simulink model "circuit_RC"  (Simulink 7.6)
settings: Solver=ode23t  StartTime=0.0  StopTime=10.0  RelTol=1e-3
InitFcn:
  | clear all, close all
  | % Durée de la simulation
  | N=10;
  | 
  | % Hauteur de l'échelon d'entrée
  | U0=5;
  | 
  | % Valeurs de la résistance R et de la capacité C
  | R=10e3;
  | C=0.1e-3;
StopFcn:
  | close all, clc
  | load circuit_RC.mat
  | plot(x(1,:),x(2,:),x(1,:),x(3,:),x(1,:),x(4,:))
  | grid
  | title('tension d''entrée, de sortie circuit et modèle théorique')
  | xlabel('temps')
  | axis([0 N -0.2 5.2])
libraries: fl_lib x6, nesl_utility x3, elec_lib x1

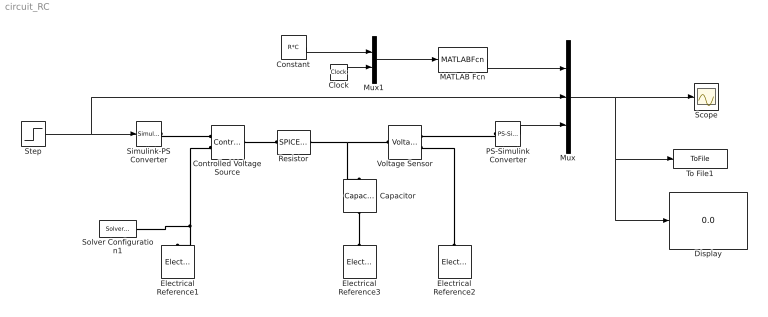
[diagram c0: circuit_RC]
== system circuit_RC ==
  Capacitor : fl_lib/Electrical/Electrical Elements/Capacitor  DialogController=NetworkEngine.DynNeDlgSource  SystemSampleTime=-1  c=C F  v0=0 V  r=0 Ohm  g=0 1/Ohm  i_Log=off  v_Log=off  vc_Log=off  LocalVarNames=|i|v|vc  LocalVarDescs=|i|v|Internal variable for voltage across capacitor term  LocalVarLogging=[0 0 0]
  Clock : Clock
  Constant : Constant  Value=R*C
  Controlled Voltage Source : fl_lib/Electrical/Electrical Sources/Controlled Voltage Source  DialogController=NetworkEngine.DynNeDlgSource  SystemSampleTime=-1  i_Log=off  v_Log=off  LocalVarNames=|current|voltage|power  LocalVarDescs=|Current (A)|Voltage (V)|Power (W)  LocalVarLogging=[0 0 0]
  Display : Display
  Electrical Reference1 : fl_lib/Electrical/Electrical Elements/Electrical Reference  DialogController=NetworkEngine.DynNeDlgSource  SystemSampleTime=-1  i_Log=off  LocalVarNames=|i  LocalVarDescs=|i  LocalVarLogging=0
  Electrical Reference2 : fl_lib/Electrical/Electrical Elements/Electrical Reference  DialogController=NetworkEngine.DynNeDlgSource  SystemSampleTime=-1  i_Log=off  LocalVarNames=|i  LocalVarDescs=|i  LocalVarLogging=0
  Electrical Reference3 : fl_lib/Electrical/Electrical Elements/Electrical Reference  DialogController=NetworkEngine.DynNeDlgSource  SystemSampleTime=-1  i_Log=off  LocalVarNames=|i  LocalVarDescs=|i  LocalVarLogging=0
  MATLAB Fcn : MATLABFcn  MATLABFcn=U0*(1-exp(-u(2)/u(1)))  Output1D=off
  Mux : Mux  Inputs=3
  Mux1 : Mux  Inputs=2
  PS-Simulink Converter : nesl_utility/PS-Simulink Converter  DialogController=NetworkEngine.DynNeUtilDlgSource  SystemSampleTime=-1  PhysicalDomain=network_engine_domain  LeftPortType=input  RightPortType=output  SubClassName=ps_output  Unit=1  AffineConversion=off
  Resistor : elec_lib/Additional Components/SPICE-Compatible Components/Passive Devices/SPICE Resistor  DialogController=NetworkEngine.DynNeDlgSource  SystemSampleTime=-1  SCALE=1  R_param=1  R=R Ohm  RSH=0 Ohm  LENGTH=1e-06 m  WIDTH=1e-06 m  NARROW=0 m  T_param=1  TC1=0 1/K  TC2=0 1/K^2  TOFFSET=0 K  TFIXED=300.15 K  TMEAS=300.15 K  LocalVarLogging=[]
  Scope : Scope
  Simulink-PS Converter : nesl_utility/Simulink-PS Converter  DialogController=NetworkEngine.DynNeUtilDlgSource  SystemSampleTime=-1  PhysicalDomain=network_engine_domain  LeftPortType=input  RightPortType=output  SubClassName=ps_input  Unit=1  AffineConversion=off  InputFilterTimeConstant=.001  UdotUserProvided=0
  Solver Configuration1 : nesl_utility/Solver Configuration  DialogController=NetworkEngine.DynNeUtilDlgSource  SystemSampleTime=-1  PhysicalDomain=network_engine_domain  LeftPortType=input  RightPortType=generic  SubClassName=solver  Accelerate=off  Profile=off  ResidualTolerance=1e-9  MaxNonlinIter=12  MaxModeIter=2  DoFixedCost=off  UseLocalSampling=off  DoDC=off  LinearAlgebra=Sparse  LocalSolverSampleTime=.001  LocalSolverChoice=NE_BACKWARD_EULER_ADVANCER  UseLocalSolver=off
  Step : Step  Time=0  After=U0  SampleTime=0
  To File1 : ToFile  Filename=circuit_RC  MatrixName=x
  Voltage Sensor : fl_lib/Electrical/Electrical Sensors/Voltage Sensor  DialogController=NetworkEngine.DynNeDlgSource  SystemSampleTime=-1  i1_Log=off  v1_Log=off  LocalVarNames=|i1|v1  LocalVarDescs=|i1|v1  LocalVarLogging=[]
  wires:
  Step/1 -> Simulink-PS Converter/1, Mux/2
  Mux/1 -> Scope/1, Display/1, To File1/1
  Clock/1 -> Mux1/2
  Constant/1 -> Mux1/1
  Mux1/1 -> MATLAB Fcn/1
  PS-Simulink Converter/1 -> Mux/3
  MATLAB Fcn/1 -> Mux/1
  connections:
  Resistor/RConn1 -- Capacitor/LConn1 -- Voltage Sensor/LConn1
  Simulink-PS Converter/RConn1 -- Controlled Voltage Source/RConn1
  Controlled Voltage Source/RConn2 -- Electrical Reference1/LConn1 -- Solver Configuration1/RConn1
  Resistor/LConn1 -- Controlled Voltage Source/LConn1
  PS-Simulink Converter/LConn1 -- Voltage Sensor/RConn1
  Electrical Reference2/LConn1 -- Voltage Sensor/RConn2
  Electrical Reference3/LConn1 -- Capacitor/RConn1
